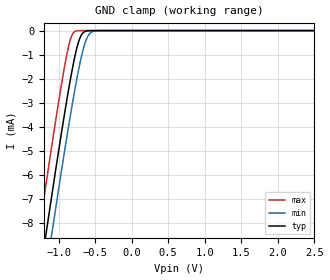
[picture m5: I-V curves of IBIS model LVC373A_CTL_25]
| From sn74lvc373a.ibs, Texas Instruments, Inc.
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[Model]   LVC373A_CTL_25
Model_type  Input
Vinl=0.7
Vinh=1.7
| variable   typ   min   max
C_comp   6.28pF   2.42pF   8.53pF
[Temperature Range]   40   100   -40
| Ambient temperature   25   85   -40
[Voltage range]   2.5   2.3   2.7
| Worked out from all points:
|   GND clamp passes 1 mA (typ) near -0.77 V on its own axis
[GND Clamp]
| LVC373A_CTL_25
|   Voltage   I(typ)   I(min)   I(max)
-5V       -90.43mA   -91.87mA   -88.61mA
-1.265V   -10.33mA   -11.92mA   -8.265mA
-1.17V    -8.383mA   -9.982mA   -6.315mA
-1.095V   -6.868mA   -8.465mA   -4.803mA
-1.07V    -6.369mA   -7.964mA   -4.307mA
-930mV    -3.652mA   -5.216mA   -1.678mA
-830mV    -1.874mA   -3.353mA   -288.1uA
-760mV    -835.1uA   -2.148mA   -17.53uA
-705mV    -284.6uA   -1.306mA   -1.254uA
-630mV    -28.82uA   -444.4uA   -32.83nA
-555mV    -1.996uA   -76.09uA   -860.6pA
2.5V      7.019pA    15.03pA    6.445pA
